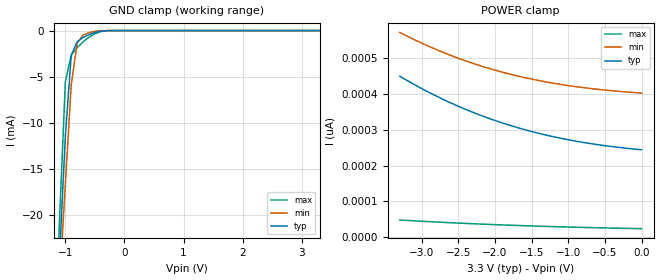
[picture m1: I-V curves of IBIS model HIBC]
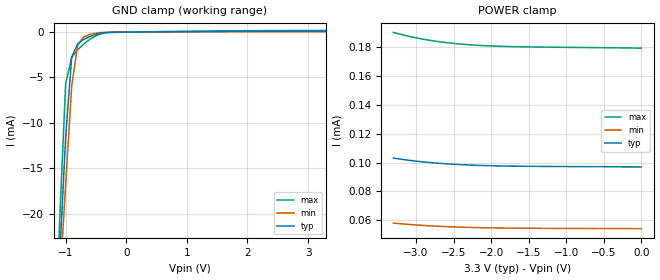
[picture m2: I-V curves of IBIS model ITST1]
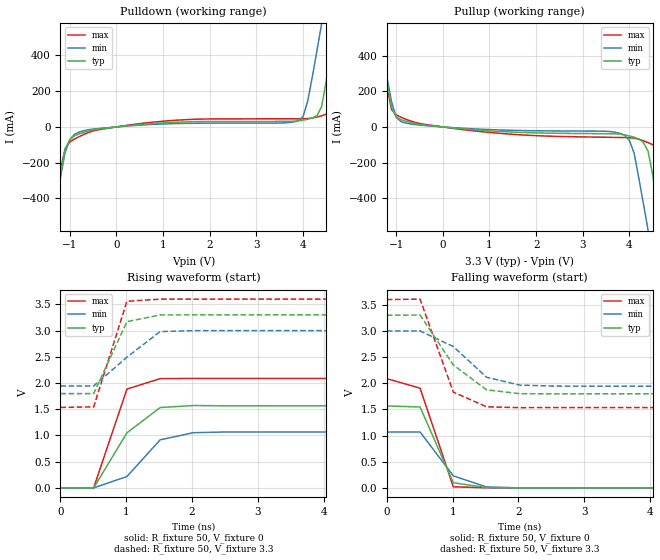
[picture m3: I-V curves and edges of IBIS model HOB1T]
[IBIS Ver]   2.1
[Comment Char]   |_char
[File name]   a5-qfp.ibs
[File Rev]   1.0
[Date]   2006/04/20 14:23
[Source]
[Notes]
[Disclaimer]
This information is for modelingpurposes only, and is not guaranteed.
[Copyright]
Copyright 2002, SEIKO EPSON Corp.
[Component]   S1D13a05
[Manufacturer]   SEIKO EPSON Corp.
| QFP5-128
| QFP5-128
[Package]
R_pkg   208.21m   190.45m   228.22m
L_pkg   3.032n   2.211n   3.786n
C_pkg   0.959p   0.823p   1.101p
[Pin] signal_name   model_name
1   VSS   GND
2   NC   NC
3   IOVDD   POWER
4   IOVDD   POWER
5   DB8   HBT2T
6   DB7   HBT2T
7   DB5   HBT2T
8   DB4   HBT2T
9   DB2   HBT2T
10   DB3   HBT2T
11   DB1   HBT2T
12   DB0   HBT2T
13   VSS   GND
14   GPO0   HOB1T
15   GPO1   HOB1T
16   GPO2   HOB1T
17   IOVDD   POWER
18   GPO3   HOB1T
19   GPIO7   US_P
20   NC   NC
21   NC   NC
22   GPIO6   US_M
23   GPIO5   HBA1T
24   GPO4   HOB1T
25   GPIO2   HBA1T
26   GPIO3   HBA1T
27   GPIO1   HBA1T
28   GPIO4   HBA1T
29   FPDAT5   HBT2T
30   GPIO0   HBA1T
31   IRQ   HOB1T
32   USBCLK   HIBC
33   IOVDD   POWER
34   DRDY   HOB1T
35   VSS   GND
36   COREVDD   POWER
37   GPO6   HOB1T
38   GPO7   HOB1T
39   COREVDD   POWER
40   FPFRAME   HBT2T
41   GPO5   HOB1T
42   FPLINE   HBT2T
43   FPSHIFT   HBT2T
44   FPDAT0   HBT2T
45   FPDAT1   HBT2T
46   FPDAT2   HBT2T
47   FPDAT3   HBT2T
48   FPDAT4   HBT2T
49   FPDAT6   HBT2T
50   VSS   GND
51   FPDAT7   HBT2T
52   IOVDD   POWER
53   FPDAT8   HBT2T
54   FPDAT12   HBT2T
55   FPDAT11   HBT2T
56   FPDAT10   HBT2T
57   FPDAT9   HBT2T
58   TESTEN   ITST1
59   FPDAT15   HBT2T
60   FPDAT14   HBT2T
61   FPDAT16   HBT2T
62   CNF6   HIBC
63   FPDAT17   HBT2T
64   GPO8   HOB1T
65   VSS   GND
66   GPO9   HOB1T
67   NC   NC
68   NC   NC
69   IOVDD   POWER
70   CLKI2   HIBC
71   PWMOUT   HOB1T
72   FPDAT13   HBT2T
73   CNF5   HIBC
74   CNF4   HIBC
75   CNF3   HIBC
76   CNF2   HIBC
77   CNF1   HIBC
78   CNF0   HIBC
79   NC   NC
80   GPO10   HOB1T
81   USBOSCO   OSCBC2
82   USBOSCI   LLIN
83   NC   NC
84   AB16   HIBC
85   AB15   HIBC
86   AB14   HIBC
87   AB12   HIBC
88   AB9   HIBC
89   NC   NC
90   AB11   HIBC
91   AB10   HIBC
92   AB6   HIBC
93   NC   NC
94   AB7   HIBC
95   AB8   HIBC
96   AB5   HIBC
97   AB4   HIBC
98   COREVDD   POWER
99   NC   NC
100   NC   NC
101   VSS   GND
102   AB3   HIBC
103   COREVDD   POWER
104   AB2   HIBC
105   AB1   HIBC
106   AB17   HIBC
107   AB0   HIBT
108   CS#   HIBC
109   M/R#   HIBT
110   BS#   HIBT
111   RD#   HIBT
112   WE0#   HIBT
113   AB13   HIBC
114   VSS   GND
115   RESET#   HIBT
116   RD/WR#   HIBT
117   WE1#   HIBT
118   CLKI   HIBC
119   WAIT#   HBT2T
120   DB15   HBT2T
121   DB14   HBT2T
122   IOVDD   POWER
123   DB12   HBT2T
124   DB11   HBT2T
125   DB10   HBT2T
126   DB13   HBT2T
127   DB9   HBT2T
128   DB6   HBT2T
| Models and submodels in the file (10): HIBC (Input), HIBT (Input), ITST1 (Input), HOB1T (Output), HBT2T (I/O), HBA1T (I/O), OSCBC2 (Output), US_M (I/O), US_P (I/O), LLIN (Input)
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[Model]   HIBC
Model_type Input
Vinh=2.0
Vinl=0.8
C_comp   5p   4p   6p
[Temperature Range] 25   85   -40
[Voltage Range]   3.3   3.0   3.6
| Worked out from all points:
|   GND clamp passes 1 mA (typ) near -0.75 V on its own axis
[GND Clamp]
-3.3V     -332.5mA   -280.8mA   -419.5mA
-1.2V     -37.95mA   -38.52mA   -38.05mA
-1.1V     -24.68mA   -27.58mA   -20.86mA
-1V       -11.47mA   -16.69mA   -5.543mA
-900mV    -2.663mA   -5.865mA   -2.666mA
-800mV    -1.216mA   -1.352mA   -1.836mA
-700mV    -746.8uA   -499.6uA   -1.216mA
-600mV    -436.7uA   -225.6uA   -715.6uA
-500mV    -208.3uA   -83.57uA   -339.6uA
-400mV    -62.86uA   -17.27uA   -100uA
-300mV    -7.502uA   -1.76uA    -9.519uA
3.3V      244pA      406.7pA    22.97pA
[POWER Clamp]
-3.3V     449.1pA    571.3pA    48.14pA
-3V       414.6pA    541.3pA    44.69pA
-2.8V     393.6pA    523.3pA    42.55pA
-2.6V     374.3pA    506.8pA    40.54pA
-2.4V     356.5pA    491.8pA    38.65pA
-2.2V     340.3pA    478.2pA    36.88pA
-2V       325.6pA    466pA      35.23pA
-1.8V     312.3pA    455.1pA    33.69pA
-1.4V     289.7pA    436.9pA    30.94pA
-1V       271.9pA    423pA      28.58pA
-500mV    255.5pA    410.5pA    26.1pA
0V        244pA      402pA      24.05pA
[Model]   ITST1
Model_type Input
Vinh=2.0
Vinl=0.8
C_comp   5p   4p   6p
[Temperature Range] 25   85   -40
[Voltage Range]   3.3   3.0   3.6
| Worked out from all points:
|   GND clamp passes 1 mA (typ) near -0.74 V on its own axis
[GND Clamp]
-3.3V     -340.8mA   -289.1mA   -427.7mA
-1.2V     -38.42mA   -39.08mA   -38.42mA
-1.1V     -24.91mA   -27.89mA   -21.04mA
-1V       -11.58mA   -16.82mA   -5.667mA
-900mV    -2.736mA   -5.931mA   -2.774mA
-800mV    -1.278mA   -1.397mA   -1.931mA
-700mV    -800uA     -536.4uA   -1.299mA
-600mV    -481.9uA   -256.4uA   -786.9uA
-500mV    -245.7uA   -108.8uA   -398.8uA
-400mV    -92.5uA    -37.21uA   -147.2uA
-300mV    -29.53uA   -16.5uA    -44.73uA
3.3V      96.95uA    54.12uA    179.2uA
[POWER Clamp]
-3.3V     103.1uA    57.94uA    190.4uA
-3.2V     102.3uA    57.46uA    189uA
-3.1V     101.6uA    57.03uA    187.8uA
-3V       101uA      56.64uA    186.7uA
-2.8V     99.95uA    55.99uA    184.8uA
-2.7V     99.51uA    55.72uA    184uA
-2.5V     98.81uA    55.27uA    182.8uA
-2.4V     98.53uA    55.09uA    182.3uA
-2.2V     98.1uA     54.81uA    181.5uA
-1.9V     97.68uA    54.53uA    180.8uA
-1.6V     97.45uA    54.37uA    180.4uA
0V        96.95uA    54.07uA    179.5uA
[Model]   HOB1T
Model_type Output
Polarity Non-Inverting
Vref=0
Vmeas=1.65
Rref=500
Cref=100pf
C_comp   5p   4p   6p
[Temperature Range] 25   85   -40
[Voltage Range]   3.3   3.0   3.6
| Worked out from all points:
|   slope of the pulldown table from 0 to 0.495 V, typ, clamps not added: 37.4 ohm
|   slope of the pullup table from 0 to 0.495 V, typ, clamps not added: 40.6 ohm
|   falling waveform, R_fixture 50, V_fixture 0: 20-80 % time 327ps typ, 411ps min, 335ps max; typ from 1.56 V to 0 V
|   falling waveform, R_fixture 50, V_fixture 3.3: 20-80 % time 610ps typ, 618ps min, 352ps max; typ from 3.3 V to 1.8 V
|   rising waveform, R_fixture 50, V_fixture 0: 20-80 % time 566ps typ, 465ps min, 336ps max; typ from 0 V to 1.56 V
|   rising waveform, R_fixture 50, V_fixture 3.3: 20-80 % time 332ps typ, 617ps min, 311ps max; typ from 1.8 V to 3.3 V
[Pullup]
-3.3V     3.845A     3.464A     4.384A
-1.4V     593.4mA    580.5mA    617.1mA
-1.1V     111.4mA    143.9mA    97.6mA
-900mV    41.07mA    30.39mA    54.95mA
1V        -21.89mA   -14.88mA   -31.01mA
3.8V      -40.63mA   -36.25mA   -59.29mA
4V        -50.66mA   -75.82mA   -60.43mA
4.1V      -57.96mA   -147.1mA   -63.03mA
4.4V      -136.9mA   -581.3mA   -88.3mA
4.7V      -606.3mA   -1.033A    -151.5mA
5V        -1.118A    -1.486A    -652.1mA
6.6V      -3.864A    -3.914A    -3.864A
[Pulldown]
-3.3V     -3.857A    -3.456A    -4.452A
-1.4V     -596.7mA   -578.9mA   -634mA
-1.1V     -123.1mA   -143.2mA   -122.5mA
-800mV    -39.04mA   -28.55mA   -54.3mA
1V        22.56mA    16.49mA    31.96mA
3.9V      34.25mA    34.83mA    45.63mA
4.1V      43.14mA    145.5mA    46.65mA
4.4V      116.3mA    580.4mA    62.61mA
4.6V      425.6mA    882.1mA    82.77mA
4.7V      595.8mA    1.033A     110mA
5V        1.107A     1.487A     623.8mA
6.6V      3.845A     3.915A     3.796A
[Falling Waveform]
R_fixture=50
V_fixture=0
V_fixture_min=0
V_fixture_max=0
0s        1.565V     1.066V     2.087V
505.1ps   1.545V     1.067V     1.905V
1.01ns    96.48mV    227.7mV    19.35mV
1.515ns   3.15mV     15.85mV    -698.8uV
2.02ns    -243.7uV   -1.251mV   281.5uV
50ns      642.4nV    19.17uV    -2.346uV
[Falling Waveform]
R_fixture=50
V_fixture=3.3
V_fixture_min=3.0
V_fixture_max=3.6
0s        3.3V       3V         3.6V
505.1ps   3.304V     3V         3.608V
1.01ns    2.349V     2.701V     1.83V
1.515ns   1.874V     2.114V     1.549V
2.02ns    1.8V       1.964V     1.533V
2.525ns   1.797V     1.945V     1.535V
50ns      1.798V     1.943V     1.534V
[Rising Waveform]
R_fixture=50
L_fixture=0
C_fixture=0
V_fixture=0
V_fixture_min=0
V_fixture_max=0
0s        0V         0V         0V
505.1ps   -62.41uV   -12.33uV   1.6mV
1.01ns    1.05V      215.6mV    1.884V
1.515ns   1.532V     916.9mV    2.084V
2.02ns    1.571V     1.052V     2.088V
2.525ns   1.565V     1.067V     2.087V
50ns      1.565V     1.066V     2.087V
[Rising Waveform]
R_fixture=50
V_fixture=3.3
V_fixture_min=3.0
V_fixture_max=3.6
0s        1.798V     1.943V     1.534V
505.1ps   1.798V     1.944V     1.545V
1.01ns    3.17V      2.493V     3.56V
1.515ns   3.299V     2.982V     3.601V
2.02ns    3.3V       2.999V     3.6V
2.525ns   3.3V       3V         3.6V
50ns      3.3V       3V         3.6V
[Ramp]
R_load=50
dV/dt_r   9.393E-1/3.226E-10   6.395E-1/3.895E-10   1.252E+0/2.445E-10
dV/dt_f   9.013E-1/4.126E-10   6.340E-1/4.890E-10   1.239E+0/3.229E-10
